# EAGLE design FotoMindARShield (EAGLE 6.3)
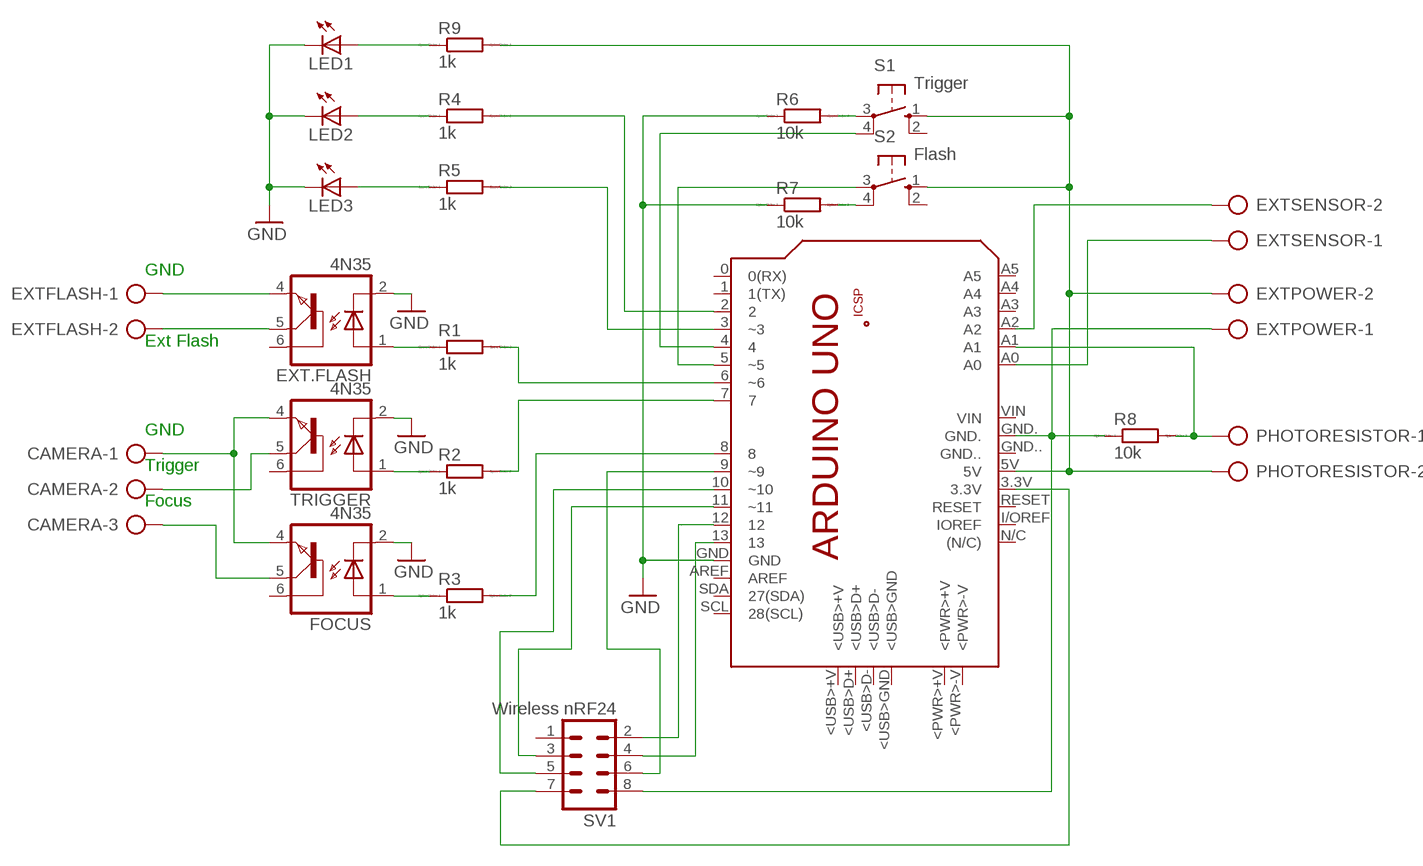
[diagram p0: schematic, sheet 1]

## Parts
CAMERA  AK300/3  [AK300/3]
EXT.FLASH  4N35  [DIL06]
EXTFLASH  AK300/2  [AK300/2]
EXTPOWER  AK300/2  [AK300/2]
EXTSENSOR  AK300/2  [AK300/2]
FOCUS  4N35  [DIL06]
LED1  LED3MM  [LED3MM]
LED2  LED3MM  [LED3MM]
LED3  LED3MM  [LED3MM]
PCB1  ARDUINO_UNO  [ARDUINO_UNO]
PHOTORESISTOR  AK300/2  [AK300/2]
R1  1k  R0204/7  [0204/7]
R2  1k  R0204/7  [0204/7]
R3  1k  R0204/7  [0204/7]
R4  1k  R0204/7  [0204/7]
R5  1k  R0204/7  [0204/7]
R6  10k  R0204/7  [0204/7]
R7  10k  R0204/7  [0204/7]
R8  10k  R0204/7  [0204/7]
R9  1k  R0204/7  [0204/7]
S1  Trigger  10-XX  [B3F-10XX]
S2  Flash  10-XX  [B3F-10XX]
SV1  Wireless nRF24  MA04-2  [MA04-2]
TRIGGER  4N35  [DIL06]

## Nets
GND: EXT.FLASH.2(C) FOCUS.2(C) LED1.K(C) LED2.K(C) LED3.K(C) PCB1.GND R6.1 R7.1 TRIGGER.2(C)
N$1: EXT.FLASH.1(A) R1.1
N$2: R2.1 TRIGGER.1(A)
N$3: FOCUS.1(A) R3.1
N$4: PCB1.6(~6) R1.2
N$5: PCB1.7 R2.2
N$6: PCB1.8 R3.2
N$7: PCB1.2 R4.2
N$8: PCB1.3(~3) R5.2
N$9: LED3.A R5.1
N$10: LED2.A R4.1
N$11: EXT.FLASH.4(EMI) EXTFLASH.1
N$12: EXT.FLASH.5(COL) EXTFLASH.2
N$13: CAMERA.1 FOCUS.4(EMI) TRIGGER.4(EMI)
N$14: CAMERA.2 TRIGGER.5(COL)
N$15: CAMERA.3 FOCUS.5(COL)
N$16: PCB1.4 S1.4(P1)
N$17: PCB1.5(~5) S2.3(P)
N$18: R6.2 S1.3(P)
N$20: R7.2 S2.4(P1)
N$21: EXTPOWER.1 PCB1.GND. R8.1 SV1.8
N$22: PCB1.A1 PHOTORESISTOR.1 R8.2
N$23: PCB1.12 SV1.2
N$24: PCB1.11(~11) SV1.3
N$25: PCB1.13 SV1.4
N$26: PCB1.10(~10) SV1.5
N$27: PCB1.9(~9) SV1.6
N$28: EXTSENSOR.1 PCB1.A0
N$29: EXTSENSOR.2 PCB1.A2
N$30: PCB1.3.3V SV1.7
N$79: EXTPOWER.2 PCB1.5V PHOTORESISTOR.2 R9.2 S1.1(S) S2.1(S)
N$92: LED1.A R9.1
Unconnected: EXT.FLASH.6(BAS) FOCUS.6(BAS) PCB1.0(0(RX)) PCB1.1(1(TX)) PCB1.+5V PCB1.<PWR>+V PCB1.<PWR>-V PCB1.<USB>+V PCB1.<USB>D+ PCB1.<USB>D- PCB1.<USB>GND PCB1.A3 PCB1.A4 PCB1.A5 PCB1.AREF PCB1.GND.. PCB1.GND_ PCB1.I/OREF(IOREF) PCB1.MISO PCB1.MOSI PCB1.N/C((N/C)) PCB1.RESET PCB1.RESET. PCB1.SCK PCB1.SCL(28(SCL)) PCB1.SDA(27(SDA)) PCB1.VIN S1.2(S1) S2.2(S1) SV1.1 TRIGGER.6(BAS)

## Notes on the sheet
- GND
- Ext Flash
- GND
- Trigger
- Focus

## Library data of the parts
CAMERA = con-ptr500:AK300/3: CONNECTOR; OC_FARNELL: unknown; OC_NEWARK: unknown
EXT.FLASH FOCUS TRIGGER = optocoupler:4N35: MOTOROLA OPTO COUPLER; MF: FAIRCHILD SEMICONDUCTOR; MPN: 4N35; OC_FARNELL: 1328375; OC_NEWARK: 72K9946
EXTFLASH EXTPOWER EXTSENSOR PHOTORESISTOR = con-ptr500:AK300/2: CONNECTOR; OC_FARNELL: unknown; OC_NEWARK: unknown
LED1-LED3 = led:LED: LED
PCB1 = E14_Arduino_published:ARDUINO_UNO: Device for representing an Arduino Uno board with a footprint in an EAGLE design. Created by Dave Young for Element14. More EAGLE documentation at: http://www.element14.com/community/community/knode/cadsoft_eagle
R1-R9 = eagle-ltspice:R: RESISTOR, European symbol; SPICEMODEL: NONE; SPICEPREFIX: R
S1 S2 = switch-omron:10-XX: OMRON SWITCH; MPN: B3F-1000; OC_FARNELL: 176432; OC_NEWARK: 36M3542
SV1 = con-lstb:MA04-2: PIN HEADER; OC_FARNELL: unknown; OC_NEWARK: unknown

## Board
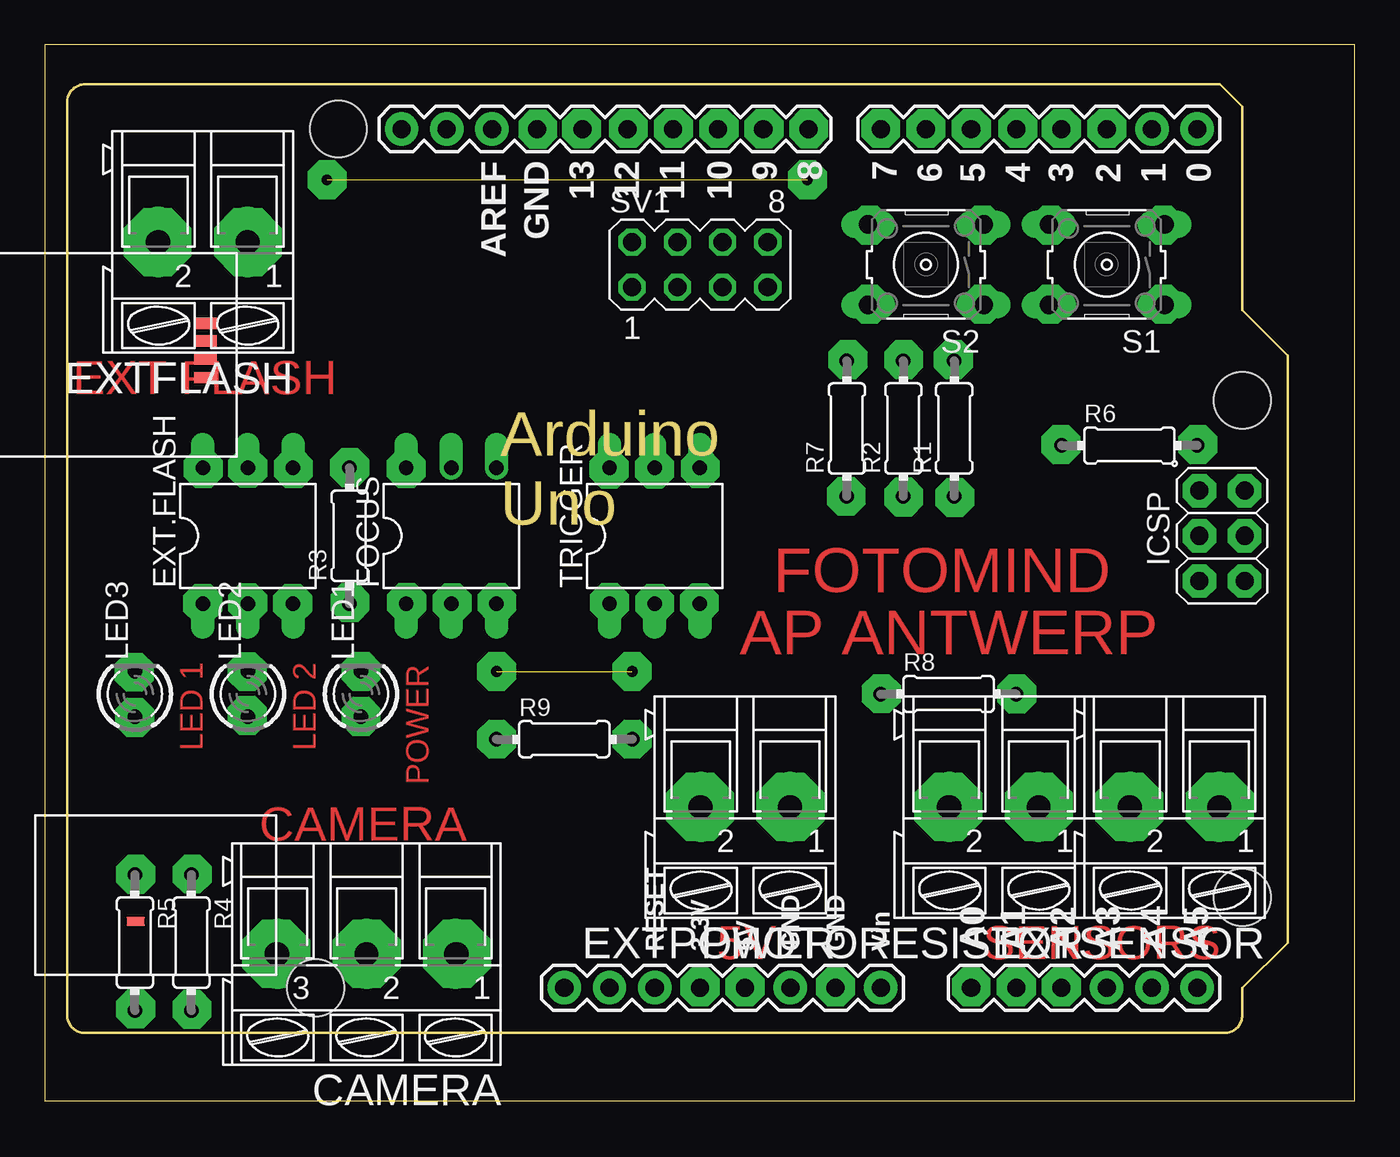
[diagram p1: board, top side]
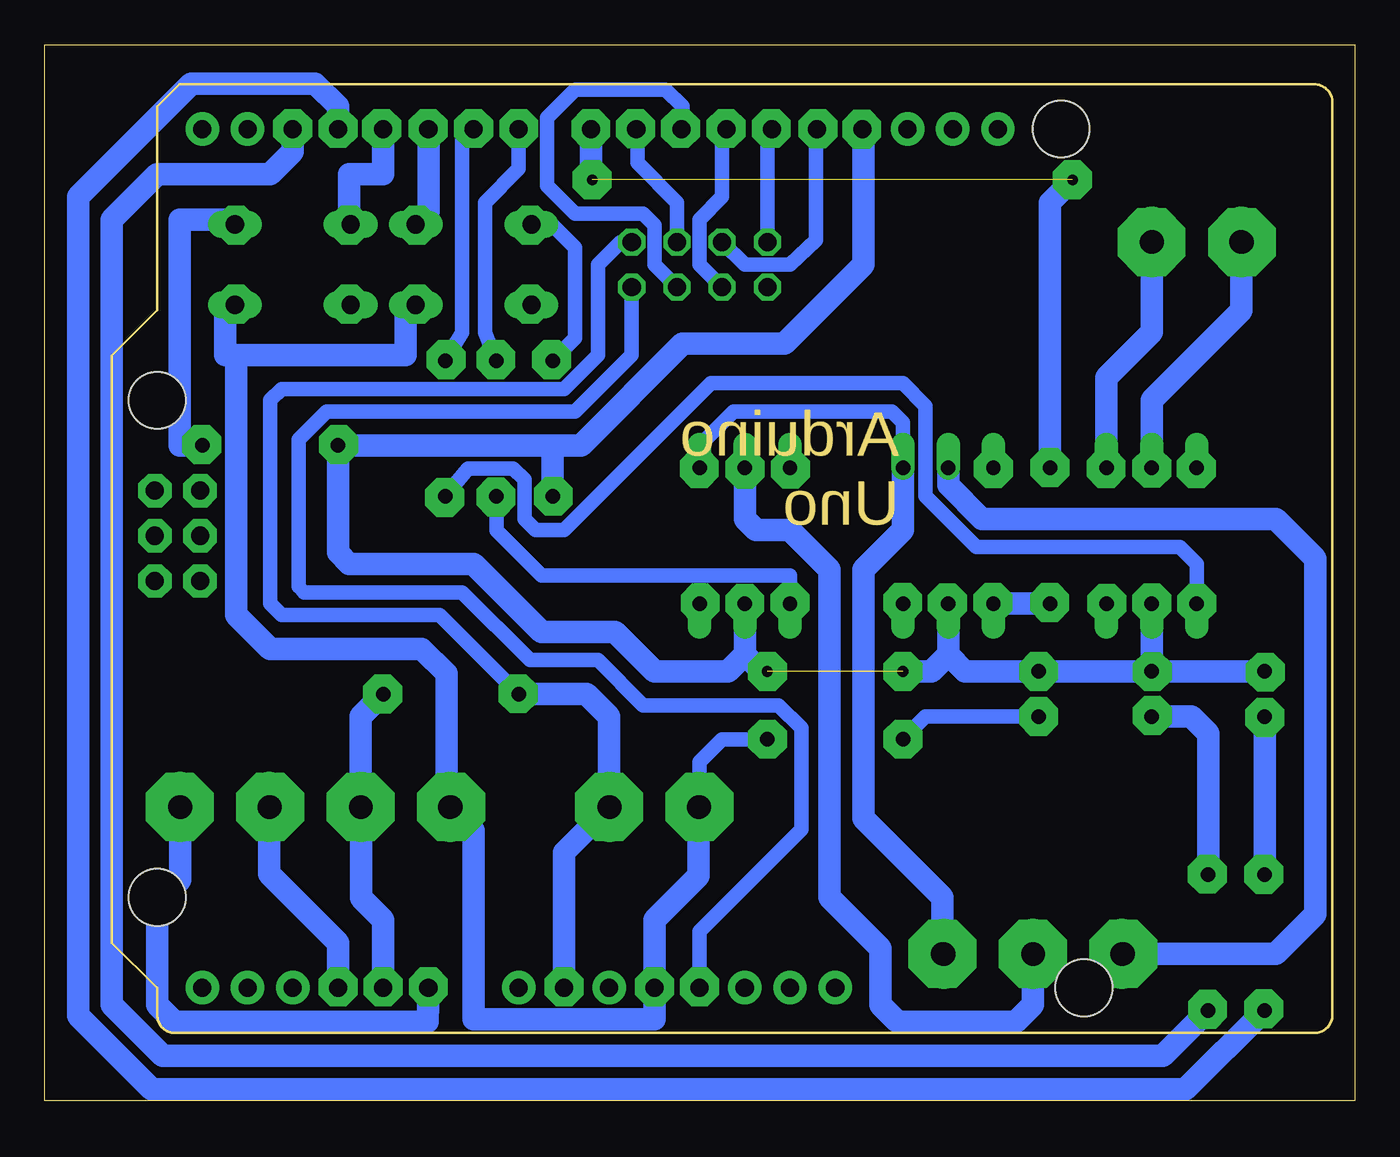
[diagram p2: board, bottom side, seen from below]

Size 73.64 x 59.36 mm. Coordinates in mm from the lower left corner, seen from the top.
Outline: 0,0 73.64,0 73.64,59.36 0,59.36 0,0
Copper layers (1*16): Top 0.035mm / dielectric 1.5mm / Bottom 0.035mm
Design rules "default": minimum track width 10mil, minimum drill 24mil, track to track 8mil, track to pad 8mil, pad to pad 8mil, via to via 8mil, smd to smd 8mil, copper to edge 40mil, drill to drill 8mil, minimum pad ring 10mil, minimum via ring 8mil, stop-mask expansion 4mil, vias tented up to drill 0mil, thermal gap 10mil

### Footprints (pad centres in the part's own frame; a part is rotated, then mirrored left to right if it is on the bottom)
AK300/3 = drill 1.321 long: 1 -5.004,0; 2 0,0; 3 5.004,0
DIL06 = drill 0.813 offset: 1 -2.54,-3.81; 2 0,-3.81; 3 2.54,-3.81; 4 2.54,3.81; 5 0,3.81; 6 -2.54,3.81
AK300/2 = drill 1.321 long: 1 -2.515,0; 2 2.489,0
LED3MM = drill 0.813 octagon: A -1.27,0; K 1.27,0
ARDUINO_UNO = drill 1.016 pad 1.88: 0 63.5,50.8; 1 60.96,50.8; 2 58.42,50.8; 3 55.88,50.8; 3.3V 35.56,2.54; 4 53.34,50.8; 5 50.8,50.8; 5V 38.1,2.54; 6 48.26,50.8; 7 45.72,50.8; 8 41.656,50.8; 9 39.116,50.8; 10 36.576,50.8; 11 34.036,50.8; 12 31.496,50.8; 13 28.956,50.8; A0 50.8,2.54; A1 53.34,2.54; A2 55.88,2.54; A3 58.42,2.54; A4 60.96,2.54; A5 63.5,2.54; AREF 23.876,50.8; GND 26.416,50.8; GND. 43.18,2.54; GND.. 40.64,2.54; I/OREF 30.48,2.54; N/C 27.94,2.54; RESET 33.02,2.54; SCL 18.796,50.8; SDA 21.336,50.8; VIN 45.72,2.54 | drill 1.016 pad 1.88 octagon: +5V 66.167,30.48; GND_ 66.167,25.4; MISO 63.627,30.48; MOSI 66.167,27.94; RESET. 63.627,25.4; SCK 63.627,27.94 | smd 1.016 x 0.508: <PWR>+V 3.861,8.814; <PWR>-V 3.861,6.274 | smd 1.27 x 0.635: <USB>+V 7.772,39.878; <USB>D+ 7.772,38.887; <USB>D- 7.772,37.871; <USB>GND 7.772,36.83 | hole 3.2: 66.04,7.62; 66.04,35.56; 15.24,50.8; 13.97,2.54
0204/7 = drill 0.813 octagon: 1 -3.81,0; 2 3.81,0
B3F-10XX = drill 1.016 long: 1 -3.251,2.261; 2 3.251,2.261; 3 -3.251,-2.261; 4 3.251,-2.261
MA04-2 = drill 1.016 octagon: 1 -3.81,-1.27; 2 -3.81,1.27; 3 -1.27,-1.27; 4 -1.27,1.27; 5 1.27,-1.27; 6 1.27,1.27; 7 3.81,-1.27; 8 3.81,1.27

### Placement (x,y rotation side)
CAMERA  18.1,8.26 180 top
EXT.FLASH  11.43,31.75 0 top
EXTFLASH  8.89,48.26 180 top
EXTPOWER  39.37,16.51 180 top
EXTSENSOR  63.5,16.51 180 top
FOCUS  22.86,31.75 0 top
LED1  17.78,22.86 90 top
LED2  11.43,22.86 90 top
LED3  5.08,22.86 90 top
PCB1  1.27,3.81 0 top
PHOTORESISTOR  53.34,16.51 180 top
R1  51.12,37.78 90 top
R2  48.26,37.78 90 top
R3  17.14,31.75 90 top
R4  8.26,8.89 270 top
R5  5.08,8.89 270 top
R6  60.96,36.83 0 top
R7  45.09,37.78 90 top
R8  50.8,22.86 0 top
R9  29.21,20.32 0 top
S1  59.69,46.99 180 top
S2  49.53,46.99 180 top
SV1  36.83,46.99 0 top
TRIGGER  34.29,31.75 0 top

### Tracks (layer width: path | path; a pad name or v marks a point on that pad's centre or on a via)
GND  (1 unrouted)
  Bottom 1.27: LED2.K EXT.FLASH.2 | LED2.K LED3.K | 27.94,54.36 PCB1.GND 27.62,54.55 27.62,46.99 32.07,42.55 37.78,42.55 43.5,36.83 45.09,36.83 | 45.09,36.83 R6.1 57.15,30.8 56.52,30.16 49.53,30.16 45.72,26.35 41.59,26.35 39.37,24.13 35.24,24.13 34.29,25.08 | R7.1 45.09,36.83 | 22.86,25.08 21.91,24.13 LED1.K LED2.K | FOCUS.2 22.86,25.08 | 22.86,25.08 23.81,24.13 25.4,24.13 | 34.29,25.08 33.34,24.13 33.02,24.13 | TRIGGER.2 34.29,25.08
N$1  (via drill 0.6 pad 2.18)
  Bottom 0.813: R1.1 49.85,35.54 47.31,35.54 46.67,34.91 46.67,32.7 46.04,32.07 44.45,32.07 36.2,40.32 25.4,40.32 24.13,39.05 24.13,33.97 21.27,31.11 9.84,31.11 8.89,30.16 v8.89,27.96 EXT.FLASH.1
N$2  (via drill 0.6 pad 2.18)
  Bottom 0.813: TRIGGER.1 v31.75,27.99 31.75,29.53 45.72,29.53 48.24,32.05 R2.1
N$3
  Bottom 1.27: FOCUS.1 R3.1
N$4
  Bottom 0.813: PCB1.6 50.16,53.98 50.16,43.18 R1.2
N$5
  Bottom 0.813: PCB1.7 46.99,52.39 48.9,50.48 48.9,43.18 R2.2
N$6  (via drill 0.6 pad 2.18)  (1 unrouted)
  Bottom 1.27: R3.2 v17.14,35.58 17.14,50.48 v15.88,51.75 | PCB1.8 42.93,51.82 42.86,51.75
N$7
  Bottom 1.27: PCB1.2 59.69,53.34 60.96,52.07 67.31,52.07 69.53,49.85 69.85,49.53 69.85,5.4 66.99,2.54 10.79,2.54 R4.2
N$8  (via drill 0.6 pad 2.18)
  Bottom 1.27: PCB1.3 v57.15,54.65 57.15,55.88 58.42,57.15 65.41,57.15 71.75,50.8 71.75,4.76 67.63,0.64 9.53,0.64 R5.2
N$9
  Bottom 1.27: LED3.A R5.1
N$10
  Bottom 1.27: LED2.A 9.21,21.59 8.26,20.64 R4.1
N$11
  Bottom 1.27: EXTFLASH.1 11.4,43.2 13.97,40.64 EXT.FLASH.4
N$12
  Bottom 1.27: EXTFLASH.2 6.4,44.4 11.43,39.37 EXT.FLASH.5
N$13
  Bottom 0.813: FOCUS.4 25.4,38.1 26.04,38.73 34.92,38.73 36.83,36.83 TRIGGER.4
  Bottom 1.27: CAMERA.1 23.18,8.33 23.18,11.43 27.62,15.88 27.62,29.84 25.4,32.07 FOCUS.4
N$14
  Bottom 1.27: TRIGGER.5 34.29,32.7 33.66,32.07 31.75,32.07 29.53,29.84 29.53,11.43 26.67,8.57 26.67,5.4 25.72,4.45 19.05,4.45 18.1,5.4 CAMERA.2
N$15  (via drill 1.3 pad 3.81)
  Bottom 1.27: CAMERA.3 v13.02,8.26 4.45,8.26 2.22,10.48 2.22,30.48 4.45,32.7 20.95,32.7 22.86,34.61 FOCUS.5
N$16
  Bottom 1.27: PCB1.4 54.61,52.07 56.52,52.07 56.52,49.96 S1.4
N$17
  Bottom 1.27: PCB1.5 52.07,49.96 S2.3
N$18
  Bottom 1.27: R6.2 66.04,36.83 66.04,49.53 63.22,49.53 S1.3
N$19  (via drill 0.6 pad 2.18)
  other vias: 17.78,21.59
N$20
  Bottom 0.813: R7.2 43.81,42.86 43.81,47.94 45.09,49.21 46.24,49.21 S2.4
N$21  (via drill 1.3 pad 3.81)
  Bottom 0.813: SV1.8 41.27,48.26 42.55,46.99 42.55,41.91 44.45,40.01 60.33,40.01 60.96,39.37 60.96,27.94 60.33,27.3 51.44,27.3 R8.1
  Bottom 1.27: PCB1.GND. 44.45,13.97 v41.91,16.51 EXTPOWER.1 41.91,16.54 41.91,21.59 43.18,22.86 R8.1
N$22
  Bottom 1.27: PCB1.A1 54.61,10.16 55.85,11.4 PHOTORESISTOR.1 55.88,16.54 55.88,21.59 R8.2
N$23
  Bottom 0.813: SV1.2 33.02,54.36 PCB1.12
N$24
  Bottom 0.813: SV1.3 36.83,46.99 36.83,49.53 35.56,50.8 35.56,54.36 PCB1.11
N$25
  Bottom 0.813: SV1.4 34.29,46.99 31.75,46.99 30.28,48.36 30.28,54.46 PCB1.13
N$26
  Bottom 0.813: SV1.5 39.37,46.99 39.37,49.21 40.01,49.85 43.81,49.85 45.4,51.44 45.4,55.24 43.81,56.83 38.73,56.83 37.78,55.88 37.78,54.67 PCB1.10
N$27
  Bottom 0.813: SV1.6 38.1,50.48 40.32,52.7 40.32,54.55 PCB1.9
N$28  (via drill 0.6 pad 2.18)
  Bottom 1.27: EXTSENSOR.1 66.02,12.41 67.31,11.11 67.31,5.4 66.36,4.45 52.12,4.45 v52.07,6.4 PCB1.A0
N$29
  Bottom 1.27: EXTSENSOR.2 61.01,12.75 57.15,8.89 PCB1.A2
N$30
  Bottom 0.813: SV1.7 40.64,41.91 43.81,38.73 57.78,38.73 59.37,37.15 59.37,28.89 59.05,28.57 50.16,28.57 46.35,24.77 42.55,24.77 40.01,22.23 32.38,22.23 31.11,20.95 31.11,15.24 36.83,9.53 PCB1.3.3V
N$31  (via drill 0.6 pad 2.18)
  other vias: 42.86,51.75
N$32  (via drill 0.6 pad 2.18)
  other vias: 25.4,24.13
N$33  (via drill 0.6 pad 2.18)
  other vias: 33.02,24.13
N$34  (via drill 0.6 pad 2.18)
  other vias: 45.05,33.97
N$35  (via drill 0.6 pad 2.18)
  other vias: 48.28,33.92
N$36  (via drill 0.6 pad 2.18)
  other vias: 51.15,33.9
N$37  (via drill 0.6 pad 2.18)
  other vias: 57.12,36.88
N$38  (via drill 0.6 pad 2.18)
  other vias: 48.28,41.65
N$39  (via drill 0.6 pad 2.18)
  other vias: 51.08,41.65
N$40  (via drill 0.6 pad 2.18)
  other vias: 45.14,41.65
N$41  (via drill 0.6 pad 2.18)
  other vias: 64.81,36.88
N$42  (via drill 0.6 pad 2.18)
  other vias: 47.04,22.88
N$43  (via drill 0.6 pad 2.18)
  other vias: 54.65,22.86
N$44  (via drill 0.6 pad 2.18)
  other vias: 5.04,24.08
N$45  (via drill 0.6 pad 2.18)
  other vias: 5.06,21.54
N$46  (via drill 0.6 pad 2.18)
  other vias: 11.38,24.11
N$47  (via drill 0.6 pad 2.18)
  other vias: 11.39,21.66
N$48  (via drill 0.6 pad 2.18)
  other vias: 17.16,28
N$49  (via drill 0.6 pad 2.18)
  other vias: 5.13,12.72
N$50  (via drill 0.6 pad 2.18)
  other vias: 5.13,5.16
N$51  (via drill 0.6 pad 2.18)
  other vias: 8.29,5.14
N$52  (via drill 0.6 pad 2.18)
  other vias: 8.3,12.73
N$53  (via drill 0.6 pad 2.18)
  other vias: 36.83,6.42
N$54  (via drill 0.6 pad 2.18)
  other vias: 44.45,6.4
N$55  (via drill 0.6 pad 2.18)
  other vias: 54.61,6.4
N$56  (via drill 0.6 pad 2.18)
  other vias: 57.15,6.4
N$57  (via drill 0.6 pad 2.18)
  other vias: 59.69,54.65
N$58  (via drill 0.6 pad 2.18)
  other vias: 54.69,54.65
N$59  (via drill 0.6 pad 2.18)
  other vias: 52.09,54.65
N$60  (via drill 0.6 pad 2.18)
  other vias: 49.53,54.65
N$61  (via drill 0.6 pad 2.18)
  other vias: 46.99,54.65
N$62  (via drill 0.6 pad 2.18)
  other vias: 42.95,54.63
N$63  (via drill 0.6 pad 2.18)
  other vias: 40.42,54.63
N$64  (via drill 0.6 pad 2.18)
  other vias: 37.9,54.65
N$65  (via drill 0.6 pad 2.18)
  other vias: 35.34,54.65
N$66  (via drill 0.6 pad 2.18)
  other vias: 32.8,54.65
N$67  (via drill 0.6 pad 2.18)
  other vias: 30.18,54.64
N$68  (via drill 0.6 pad 2.18)
  other vias: 27.72,54.61
N$69  (via drill 0.6 pad 2.18)
  other vias: 11.41,27.98
N$70  (via drill 0.6 pad 2.18)
  other vias: 13.95,27.96
N$71  (via drill 0.6 pad 2.18)
  other vias: 20.36,27.99
N$72  (via drill 0.6 pad 2.18)
  other vias: 22.89,27.98
N$73  (via drill 0.6 pad 2.18)
  other vias: 25.42,27.99
N$74  (via drill 0.6 pad 2.18)
  other vias: 34.29,27.96
N$75  (via drill 0.6 pad 2.18)
  other vias: 36.8,27.98
N$76  (via drill 0.6 pad 2.18)
  other vias: 36.85,35.52
N$77  (via drill 0.6 pad 2.18)
  other vias: 34.27,35.51
N$78  (via drill 0.6 pad 2.18)
  other vias: 31.73,35.51
N$79  (via drill 0.6 pad 2.18)
  Bottom 0.813: R9.2 35.56,20.32 36.83,19.05 36.83,16.56 EXTPOWER.2
  Bottom 1.27: S2.1 53.06,44.73 53.34,44.45 53.34,41.91 62.87,41.91 | 62.87,41.91 63.5,41.91 63.5,44.17 S1.1 | EXTPOWER.2 36.88,12.65 39.37,10.16 PCB1.5V v39.37,6.42 39.37,4.57 49.53,4.57 49.53,15.19 PHOTORESISTOR.2 51.05,16.71 51.05,24 52.45,25.4 60.96,25.4 62.87,27.3 62.87,41.91
N$80  (via drill 0.6 pad 2.18)
  other vias: 20.32,35.52
N$81  (via drill 0.6 pad 2.18)
  other vias: 13.99,35.52
N$82  (via drill 0.6 pad 2.18)
  other vias: 11.41,35.54
N$83  (via drill 0.6 pad 2.18)
  other vias: 8.91,35.52
N$84  (via drill 0.6 pad 2.18)
  other vias: 46.35,49.21
N$85  (via drill 0.6 pad 2.18)
  other vias: 46.35,44.77
N$86  (via drill 0.6 pad 2.18)
  other vias: 52.7,44.77
N$87  (via drill 0.6 pad 2.18)
  other vias: 52.7,49.21
N$88  (via drill 0.6 pad 2.18)
  other vias: 56.52,49.21
N$89  (via drill 0.6 pad 2.18)
  other vias: 56.52,44.77
N$90  (via drill 0.6 pad 2.18)
  other vias: 62.87,44.77
N$91  (via drill 0.6 pad 2.18)
  other vias: 62.87,49.21
N$92
  Bottom 0.813: LED1.A 24.13,21.59 R9.1
N$93  (via drill 0.6 pad 2.18)
  other vias: 17.78,24.13
N$94  (via drill 0.6 pad 2.18)
  other vias: 25.4,20.32
N$95  (via drill 0.6 pad 2.18)
  other vias: 33.02,20.32
N$96  (via drill 1.3 pad 3.81)
  other vias: 6.35,48.26
N$97  (via drill 1.3 pad 3.81)
  other vias: 11.43,48.26
N$98  (via drill 1.3 pad 3.81)
  other vias: 18.1,8.26
N$99  (via drill 1.3 pad 3.81)
  other vias: 23.18,8.26
N$100  (via drill 1.3 pad 3.81)
  other vias: 36.83,16.51
N$101  (via drill 1.3 pad 3.81)
  other vias: 50.8,16.51
N$102  (via drill 1.3 pad 3.81)
  other vias: 55.88,16.51
N$103  (via drill 1.3 pad 3.81)
  other vias: 60.96,16.51
N$104  (via drill 1.3 pad 3.81)
  other vias: 66.04,16.51

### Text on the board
Top: EXT FLASH | FOTOMIND | AP ANTWERP | LED 1 | LED 2 | POWER | CAMERA | 5V | SENSORS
